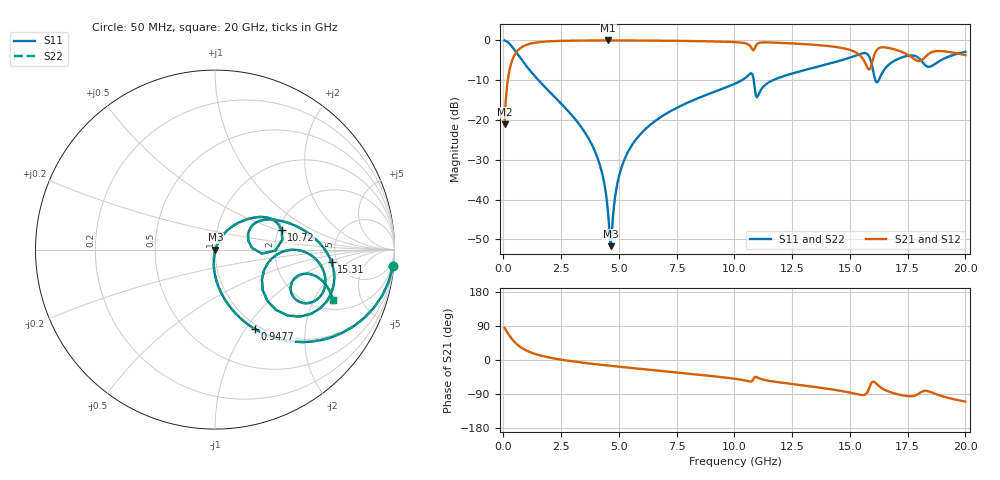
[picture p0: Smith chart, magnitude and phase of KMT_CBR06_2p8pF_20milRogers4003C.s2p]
! Data measured by Modelithics Inc. support@modelithics.com 813-866-6335
! KEMET CBR0603 2.8pF, Pad Width= 0.851mm, Pad Length= 0.64mm, Pad Gap= 0.62mm, 20mil Rogers 4003C substrate Data, January 2022
# hz S ma R 50
! 2 Port Network Data from SP1.SP block
! freq  magS11  angS11  magS21  angS21  magS12  angS12  magS22  angS22
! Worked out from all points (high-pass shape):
!   401 points, 50 MHz to 20 GHz, reference 50 ohm
!   highest |S21| = -0.02 dB at 4.539 GHz (marker M1); lowest = -21.0 dB at 50 MHz (marker M2)
!   |S21| within 3 dB of the highest: 553.5 MHz to 15.26 GHz (14.71 GHz wide, 186 % of centre); 16.1 GHz to 17.3 GHz (1.198 GHz wide, 7.17 % of centre)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
!   lowest |S11| = -51.7 dB at 4.638 GHz (marker M3), VSWR 1.01, Z = 50.2 - j0.0911 ohm
!   |S11| at or under -10 dB: 1.514 GHz to 10.33 GHz (8.812 GHz wide, 149 % of centre); 10.84 GHz to 11.67 GHz (836.4 MHz wide, 7.43 % of centre); 16.1 GHz to 16.24 GHz (143.4 MHz wide, 0.887 % of centre)
!   |S22| runs from -51.7 to 0.0 dB; largest |S21 - S12| = 0
!   S11 on the Smith chart (normalised r, x): 50 MHz: 1, -22; 947.8 MHz: 0.94, -1.10; 10.72 GHz: 2.09, +0.53; 15.31 GHz: 4.48, -1.10; 20 GHz: 2.47, -2.89
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5e7  0.996 -5.3  0.08869 84.7  0.08869 84.7  0.996 -5.3
3.4925e8  0.8475 -33.2  0.5299 56.8  0.5299 56.8  0.8475 -33.2
9.4775e8  0.4943 -63.4  0.8681 26.5  0.8681 26.5  0.4943 -63.4
1.795625e9  0.259 -80.6  0.9642 9.0  0.9642 9.0  0.259 -80.6
3.391625e9  0.07958 -95.1  0.9945 -6.7  0.9945 -6.7  0.07958 -95.1
4.189625e9  0.02629 -97.1  0.9971 -12.4  0.9971 -12.4  0.02629 -97.1
4.53875e9  0.006352 -81.0  0.9973 -14.8  0.9973 -14.8  0.006352 -81.0
4.6385e9  0.002598 -20.4  0.9972 -15.4  0.9972 -15.4  0.002598 -20.4
4.93775e9  0.01625 63.2  0.997 -17.3  0.997 -17.3  0.01625 63.2
5.286875e9  0.03434 65.8  0.9964 -19.5  0.9964 -19.5  0.03434 65.8
6.73325e9  0.105 59.9  0.991 -28.3  0.991 -28.3  0.105 59.9
1.0025e10  0.2856 38.8  0.95 -49.6  0.95 -49.6  0.2856 38.8
1.072325e10  0.3871 16.3  0.8169 -57.0  0.8169 -57.0  0.3871 16.3
1.10225e10  0.2019 24.4  0.9172 -47.2  0.9172 -47.2  0.2019 24.4
1.336662e10  0.4484 18.5  0.8835 -70.2  0.8835 -70.2  0.4484 18.5
1.531175e10  0.6531 -6.2  0.6911 -90.2  0.6911 -90.2  0.6531 -6.2
1.586038e10  0.6034 -38.2  0.4342 -69.8  0.4342 -69.8  0.6034 -38.2
1.615962e10  0.2964 -23.1  0.7545 -63.3  0.7545 -63.3  0.2964 -23.1
1.670825e10  0.5023 -1.6  0.7992 -83.8  0.7992 -83.8  0.5023 -1.6
1.795512e10  0.607 -29.2  0.5493 -89.7  0.5493 -89.7  0.607 -29.2
1.875312e10  0.521 -14.9  0.7332 -90.6  0.7332 -90.6  0.521 -14.9
2e10  0.718 -23.3  0.6535 -109.8  0.6535 -109.8  0.718 -23.3
